| IBIS file stm32mp211_213_215_tfbga289.ibs
[IBIS ver] 5.1
[File name] stm32mp211_213_215_tfbga289.ibs
[File Rev] 0.4
[Date] 09-10-2025
[Source] Data Created at STMicroelectronics
[Notes]  File originated from ELDO simulations.
[Disclaimer]  This information is for modeling purpose only and is
   not guaranted. The information is subject to change without
   notice.
[Copyright] Copyright 2025 STMicroelectronics Inc.
|   Component stm32mp211_213_215_tfbga289
[Component] stm32mp211_213_215_tfbga289
[Manufacturer] STMicroelectronics
[Package]
| variable   typ   min   max
R_pkg  0  NA  NA
L_pkg  0  NA  NA
C_pkg  0  NA  NA
[Pin]   signal_name   model_name
A1  VSS  gnd
A2  CSI_D1P  DPHY_IBIS_L1
A3  CSI_CKP  DPHY_IBIS_L1
A4  PD11  io8_tt_i3c
A5  PD2  io8_tt
A6  PB7  io8_tt
A7  PD15  io8_tt_i3c
A8  PB10  io8_tt
A9  PE5  io8_tt
A10  PE2  io8_tt
A11  PE7  io8_tt
A12  PE11  io8_tt
A13  PE10  io8_tt
A14  PD13  io8_tt
A15  DDR_DQ11  mal4drv27_PAD
A16  DDR_DQ9  mal4drv27_PAD
A17  VSS  gnd
B1  CSI_D0P  DPHY_IBIS_L1
B2  CSI_D1N  DPHY_IBIS_L1
B3  CSI_CKN  DPHY_IBIS_L1
B4  PD10  io8_tt_i3c
B5  PD3  io8_tt
B6  PD8  io8_tt
B7  PB1  io8_tt
B8  PD0  io8_tt
B9  PE4  io8_tt
B10  PE1  io8_tt
B11  PE6  io8_tt
B12  PE9  io8_tt
B13  PE12  io8_tt
B14  PB12  io8_tt
B15  DDR_DQ10  mal4drv27_PAD
B16  DDR_DQS1N  mal4drv27_PAD
B17  DDR_DQS1P  mal4drv27_PAD
C1  CSI_D0N  DPHY_IBIS_L1
C2  VDDCSI  nc
C3  CSI_REXT  nc
C4  VDDA18CSI  power
C5  PD4  io8_tt
C6  PD1  io8_tt
C7  PB3  io8_tt
C8  PB2  io8_tt
C9  PE3  io8_tt
C10  PE0  io8_tt
C11  PE8  io8_tt
C12  PE13  io8_tt
C13  PD7  io8_tt
C14  PD12  io8_tt
C15  DDR_DQ8  mal4drv27_PAD
C16  DDR_DQ15  mal4drv27_PAD
C17  DDR_DQM1  mal4drv27_PAD
D1  PI6  io8_tt
D2  PG2  io8_tt_i3c
D3  PB15  io8_tt
D4  PI5  io8_tt
D5  PB11  io8_tt
D6  PB5  io8_tt_i3c
D7  PD9  io8_tt
D8  PD6  io8_tt
D9  PD5  io8_tt
D10  VDDIO1  power
D11  PE15  io8_tt
D12  PE14  io8_tt
D13  PB13  io8_tt
D14  PD14  io8_tt
D15  DDR_DQ14  mal4drv27_PAD
D16  DDR_DQ13  mal4drv27_PAD
D17  DDR_DQ12  mal4drv27_PAD
E1  PI1  io8_tt_i3c
E2  PA7  io8_tt
E3  PF5  io8_tt
E4  PI0  io8_tt
E5  PB6  io8_tt
E6  PB9  io8_tt
E7  VDDCORE  nc
E8  VDDIO3  power
E9  VDDIO3  power
E10  VDDIO2  power
E11  VDDCPU  nc
E12  VSS  gnd
E13  VDDA18PLL1  nc
E14  PB14  io8_tt
E15  DDR_RESETN  nc
E16  DDR_A9  mal4drv20_PAD
E17  DDR_A20  mal4drv20_PAD
F1  PG14  io8_tt
F2  PG15  io8_tt
F3  PF6  io8_tt
F4  PI4  io8_tt
F5  VDDA18PLL2  nc
F6  VDDCORE  nc
F7  VSS  gnd
F8  VDDCORE  nc
F9  VSS  gnd
F10  VDDCPU  nc
F11  VSS  gnd
F12  VDDCPU  nc
F13  VSS  gnd
F14  DDR_ZQ  nc
F15  DDR_A0  mal4drv20_PAD
F16  DDR_A11  mal4drv20_PAD
F17  DDR_A21  mal4drv20_PAD
G1  PG12  io8_tt
G2  PG11  io8_tt
G3  PG10  io8_tt
G4  PG9  io8_tt
G5  V08CAP  nc
G6  VSS  gnd
G7  VDDCORE  nc
G8  VSS  gnd
G9  VDDCORE  nc
G10  VSS  gnd
G11  VDDCPU  nc
G12  VSS  gnd
G13  VDDA18DDR  nc
G14  DDR_A7  mal4drv20_PAD
G15  DDR_A1  mal4drv20_PAD
G16  DDR_A10  mal4drv20_PAD
G17  DDR_A22  mal4drv20_PAD
H1  PF11  io8_tt
H2  PA5  io8_tt
H3  PH5  io8_tt
H4  PG8  io8_tt
H5  VBAT  power
H6  VDDCORE  nc
H7  VSS  gnd
H8  VDDCORE  nc
H9  VSS  gnd
H10  VDDCPU  nc
H11  VSS  gnd
H12  VDDQDDR  power
H13  VSS  gnd
H14  DDR_A8  mal4drv20_PAD
H15  DDR_A6  mal4drv20_PAD
H16  DDR_A25  mal4drv20_PAD
H17  DDR_A23  mal4drv20_PAD
J1  PG7  io8_tt
J2  PZ0  io8_tt_i3c_tamp
J3  PZ3  io8_tt_i3c_tamp
J4  PZ1  io8_tt_i3c_tamp
J5  VSSAON  nc
J6  VSS  gnd
J7  VDDCORE  nc
J8  VSS  gnd
J9  VDDCORE  nc
J10  VSS  gnd
J11  VDDCPU  nc
J12  VSS  gnd
J13  VDDQDDR  power
J14  DDR_A3  mal4drv20_PAD
J15  DDR_A26  mal4drv20_PAD
J16  DDR_A5  mal4drv20_PAD
J17  DDR_A13  mal4drv20_PAD
K1  PA10  io8_tt
K2  PF4  io8_tt
K3  PG5  io8_tt
K4  PA0  io8_tt
K5  VDDA18AON  power
K6  VDDCORE  nc
K7  VSS  gnd
K8  VDDCORE  nc
K9  VSS  gnd
K10  VDDCORE  nc
K11  VSS  gnd
K12  VDDQDDR  power
K13  VSS  gnd
K14  DDR_A27  mal4drv20_PAD
K15  DDR_A14  mal4drv20_PAD
K16  DDR_A4  mal4drv20_PAD
K17  DDR_A2  mal4drv20_PAD
L1  PA1  io8_tt_i3c
L2  PF13  io8_tt
L3  PF15  io8_tt
L4  PI8  io8_tt
L5  PG3  io8_tt
L6  VSSA  nc
L7  VDD  power
L8  VSS  gnd
L9  VDD  power
L10  VSS  gnd
L11  VDDCORE  nc
L12  VSS  gnd
L13  VDDQDDR  power
L14  DDR_VREF  nc
L15  DDR_A16  mal4drv20_PAD
L16  DDR_A28  mal4drv20_PAD
L17  DDR_A15  mal4drv20_PAD
M1  PG4  io8_tt
M2  PG13  io8_tt_i3c
M3  PC13  io8_tt
M4  PF10  io8_tt
M5  PF8  io8_tt
M6  VDDA18ADC  power
M7  VSS  gnd
M8  VDD  power
M9  VSS  gnd
M10  VDD  power
M11  VSS  gnd
M12  PF3  io8_tt
M13  PA2  io8_tt_i3c
M14  PA3  io8_tt_i3c
M15  DDR_A31  mal4drv20_PAD
M16  DDR_A17  mal4drv20_PAD
M17  DDR_A29  mal4drv20_PAD
N1  PF12  io8_tt
N2  NJTRST  io8_tt
N3  JTCK_SWCLK  io8_tt
N4  JTMS_SWDIO  io8_tt
N5  PC3  io8_tt
N6  PF7  io8_tt
N7  PC4  io8_tt
N8  PC10  io8_tt
N9  PC0  io8_tt
N10  PH9  io8_tt
N11  PF2  io8_tt_i3c
N12  PH8  io8_tt
N13  PA9  io8_tt
N14  PH4  io8_tt
N15  DDR_A12  mal4drv20_PAD
N16  DDR_A18  mal4drv20_PAD
N17  DDR_A30  mal4drv20_PAD
P1  OSC32_IN  isudq_v18
P2  OSC32_OUT  isudq_v18
P3  JTDI  io8_tt
P4  JTDO_TRACESWO  io8_tt
P5  PC5  io8_tt_i3c
P6  PC6  io8_tt_i3c
P7  PC7  io8_tt
P8  PC9  io8_tt
P9  PA14  io8_tt
P10  PA11  io8_tt
P11  PF0  io8_tt_i3c
P12  PH7  io8_tt
P13  VDDA18USB  power
P14  VDD33USB  power
P15  DDR_DQM0  mal4drv27_PAD
P16  DDR_DQ5  mal4drv27_PAD
P17  DDR_DQ4  mal4drv27_PAD
R1  PWR_CPUON  io8_tt
R2  NRST  nc
R3  PWR_ON  io8_tt
R4  PWR_LP  io8_tt
R5  BOOT3  isudq_tt
R6  PG0  io8_tt_i3c
R7  PC12  io8_tt_i3c
R8  PC8  io8_tt
R9  PA13  io8_tt
R10  PA15  io8_tt_i3c
R11  PH11  io8_tt
R12  PA8  io8_tt_i3c
R13  USBH_HS_TXRTUNE  nc
R14  OTG_TXRTUNE  nc
R15  DDR_DQ3  mal4drv27_PAD
R16  DDR_DQ7  mal4drv27_PAD
R17  DDR_DQ6  mal4drv27_PAD
T1  PDR_ON  nc
T2  OSC_IN  isudq_v18
T3  BOOT2  isudq_tt
T4  BOOT0  isudq_tt
T5  VREFN  nc
T6  ANA0  nc
T7  PF9  io8_tt
T8  PF1  io8_tt
T9  PH12  io8_tt
T10  PC1  io8_tt_i3c
T11  PG1  io8_tt_i3c
T12  PA6  io8_tt
T13  USBH_HS_DP  USB2_HS_IBIS
T14  OTG_HSDP  USB2_HS_IBIS
T15  DDR_DQ2  mal4drv27_PAD
T16  DDR_DQS0N  mal4drv27_PAD
T17  DDR_DQS0P  mal4drv27_PAD
U1  VSS  gnd
U2  OSC_OUT  isudq_v18
U3  BOOT1  isudq_tt
U4  NRSTC1MS  io8_tt
U5  VREFP  nc
U6  ANA1  nc
U7  PC11  io8_tt
U8  PC2  io8_tt
U9  PH13  io8_tt
U10  PH10  io8_tt
U11  PA12  io8_tt_i3c
U12  PA4  io8_tt
U13  USBH_HS_DM  USB2_HS_IBIS
U14  OTG_HSDM  USB2_HS_IBIS
U15  DDR_DQ1  mal4drv27_PAD
U16  DDR_DQ0  mal4drv27_PAD
U17  VSS  gnd
[Package Model]   503-fctfbga-14x14-289-240814
[Pin Mapping]   pulldown_ref   pullup_ref   | Comment
A1  gnd  nc
A2  gnd  VDDA18CSI
A3  gnd  VDDA18CSI
A4  gnd  vddio3
A5  gnd  vddio3
A6  gnd  vdd
A7  gnd  vdd
A8  gnd  vdd
A9  gnd  vddio1
A10  gnd  vddio1
A11  gnd  vddio1
A12  gnd  vddio2
A13  gnd  vddio2
A14  gnd  vdd
A15  gnd  vddqddr
A16  gnd  vddqddr
A17  gnd  nc
B1  gnd  VDDA18CSI
B2  gnd  VDDA18CSI
B3  gnd  VDDA18CSI
B4  gnd  vddio3
B5  gnd  vddio3
B6  gnd  vddio3
B7  gnd  vdd
B8  gnd  vddio3
B9  gnd  vddio1
B10  gnd  vddio1
B11  gnd  vddio1
B12  gnd  vddio1
B13  gnd  vddio2
B14  gnd  vdd
B15  gnd  vddqddr
B16  gnd  vddqddr
B17  gnd  vddqddr
C1  gnd  VDDA18CSI
C2  nc  nc
C3  nc  nc
C4  nc  VDDA18CSI
C5  gnd  vddio3
C6  gnd  vddio3
C7  gnd  vdd
C8  gnd  vdd
C9  gnd  vddio1
C10  gnd  vddio1
C11  gnd  vddio1
C12  gnd  vddio2
C13  gnd  vddio3
C14  gnd  vdd
C15  gnd  vddqddr
C16  gnd  vddqddr
C17  gnd  vddqddr
D1  gnd  vdd
D2  gnd  vdd
D3  gnd  vdd
D4  gnd  vdd
D5  gnd  vdd
D6  gnd  vdd
D7  gnd  vddio3
D8  gnd  vddio3
D9  gnd  vddio3
D10  nc  vddio1
D11  gnd  vddio2
D12  gnd  vddio2
D13  gnd  vdd
D14  gnd  vdd
D15  gnd  vddqddr
D16  gnd  vddqddr
D17  gnd  vddqddr
E1  gnd  vdd
E2  gnd  vdd
E3  gnd  vdd
E4  gnd  vdd
E5  gnd  vdd
E6  gnd  vdd
E7  nc  nc
E8  nc  vddio3
E9  nc  vddio3
E10  nc  vddio2
E11  nc  nc
E12  gnd  nc
E13  nc  nc
E14  gnd  vdd
E15  nc  nc
E16  gnd  vddqddr
E17  gnd  vddqddr
F1  gnd  vdd
F2  gnd  vdd
F3  gnd  vdd
F4  gnd  vdd
F5  nc  nc
F6  nc  nc
F7  gnd  nc
F8  nc  nc
F9  gnd  nc
F10  nc  nc
F11  gnd  nc
F12  nc  nc
F13  gnd  nc
F14  nc  nc
F15  gnd  vddqddr
F16  gnd  vddqddr
F17  gnd  vddqddr
G1  gnd  vdd
G2  gnd  vdd
G3  gnd  vdd
G4  gnd  vdd
G5  nc  nc
G6  gnd  nc
G7  nc  nc
G8  gnd  nc
G9  nc  nc
G10  gnd  nc
G11  nc  nc
G12  gnd  nc
G13  nc  nc
G14  gnd  vddqddr
G15  gnd  vddqddr
G16  gnd  vddqddr
G17  gnd  vddqddr
H1  gnd  vdd
H2  gnd  vdd
H3  gnd  vdd
H4  gnd  vdd
H5  nc  vsw
H6  nc  nc
H7  gnd  nc
H8  nc  nc
H9  gnd  nc
H10  nc  nc
H11  gnd  nc
H12  nc  vddqddr
H13  gnd  nc
H14  gnd  vddqddr
H15  gnd  vddqddr
H16  gnd  vddqddr
H17  gnd  vddqddr
J1  gnd  vdd
J2  gnd  vdd  | Depending on IO usage
| J2  gnd  vsw  | Depending on IO usage
J3  gnd  vdd  | Depending on IO usage
| J3  gnd  vsw  | Depending on IO usage
J4  gnd  vdd  | Depending on IO usage
| J4  gnd  vsw  | Depending on IO usage
J5  nc  nc
J6  gnd  nc
J7  nc  nc
J8  gnd  nc
J9  nc  nc
J10  gnd  nc
J11  nc  nc
J12  gnd  nc
J13  nc  vddqddr
J14  gnd  vddqddr
J15  gnd  vddqddr
J16  gnd  vddqddr
J17  gnd  vddqddr
K1  gnd  vdd
K2  gnd  vdd
K3  gnd  vdd
K4  gnd  vdd
K5  nc  vdda18aon
K6  nc  nc
K7  gnd  nc
K8  nc  nc
K9  gnd  nc
K10  nc  nc
K11  gnd  nc
K12  nc  vddqddr
K13  gnd  nc
K14  gnd  vddqddr
K15  gnd  vddqddr
K16  gnd  vddqddr
K17  gnd  vddqddr
L1  gnd  vdd
L2  gnd  vdd
L3  gnd  vdd
L4  gnd  vdd
L5  gnd  vdd
L6  nc  nc
L7  nc  vdd
L8  gnd  nc
L9  nc  vdd
L10  gnd  nc
L11  nc  nc
L12  gnd  nc
L13  nc  vddqddr
L14  nc  nc
L15  gnd  vddqddr
L16  gnd  vddqddr
L17  gnd  vddqddr
M1  gnd  vdd
M2  gnd  vdd
M3  gnd  vdd  | Depending on IO usage
| M3  gnd  vsw  | Depending on IO usage
M4  gnd  vdd
M5  gnd  vdd
M6  nc  vdda18adc
M7  gnd  nc
M8  nc  vdd
M9  gnd  nc
M10  nc  vdd
M11  gnd  nc
M12  gnd  vdd
M13  gnd  vdd
M14  gnd  vdd
M15  gnd  vddqddr
M16  gnd  vddqddr
M17  gnd  vddqddr
N1  gnd  vdd
N2  gnd  vdd
N3  gnd  vdd
N4  gnd  vdd
N5  gnd  vdd
N6  gnd  vdd
N7  gnd  vdd
N8  gnd  vdd
N9  gnd  vdd
N10  gnd  vdd
N11  gnd  vdd
N12  gnd  vdd
N13  gnd  vdd
N14  gnd  vdd
N15  gnd  vddqddr
N16  gnd  vddqddr
N17  gnd  vddqddr
P1  gnd  vdd  | Depending on IO usage
| P1  gnd  vsw  | Depending on IO usage
P2  gnd  vdd  | Depending on IO usage
| P2  gnd  vsw  | Depending on IO usage
P3  gnd  vdd
P4  gnd  vdd
P5  gnd  vdd
P6  gnd  vdd
P7  gnd  vdd
P8  gnd  vdd
P9  gnd  vdd
P10  gnd  vdd
P11  gnd  vdd
P12  gnd  vdd
P13  nc  vdda18usb
P14  nc  VDD33USB
P15  gnd  vddqddr
P16  gnd  vddqddr
P17  gnd  vddqddr
R1  gnd  vdd
R2  nc  nc
R3  gnd  vdd
R4  gnd  vdd
R5  gnd  vdd
R6  gnd  vdd
R7  gnd  vdd
R8  gnd  vdd
R9  gnd  vdd
R10  gnd  vdd
R11  gnd  vdd
R12  gnd  vdd
R13  nc  nc
R14  nc  nc
R15  gnd  vddqddr
R16  gnd  vddqddr
R17  gnd  vddqddr
T1  nc  nc
T2  gnd  vdda18aon
T3  gnd  vdd
T4  gnd  vdd
T5  nc  nc
T6  nc  nc
T7  gnd  vdd
T8  gnd  vdd
T9  gnd  vdd
T10  gnd  vdd
T11  gnd  vdd
T12  gnd  vdd
T13  gnd  VDD33USB
T14  gnd  VDD33USB
T15  gnd  vddqddr
T16  gnd  vddqddr
T17  gnd  vddqddr
U1  gnd  nc
U2  gnd  vdda18aon
U3  gnd  vdd
U4  gnd  vdd
U5  nc  nc
U6  nc  nc
U7  gnd  vdd
U8  gnd  vdd
U9  gnd  vdd
U10  gnd  vdd
U11  gnd  vdd
U12  gnd  vdd
U13  gnd  VDD33USB
U14  gnd  VDD33USB
U15  gnd  vddqddr
U16  gnd  vddqddr
U17  gnd  nc
[Diff Pin]  inv_pin  vdiff  tdelay_typ  tdelay_min  tdelay_max
B3  A3  NA  NA  NA  NA
C1  B1  NA  NA  NA  NA
B2  A2  NA  NA  NA  NA
T17  T16  NA  NA  NA  NA
B17  B16  NA  NA  NA  NA
T13  U13  NA  NA  NA  NA   |USBH_HS_DP _DM
T14  U14  NA  NA  NA  NA   |USBH_HS_DP _DM
K16  J16  NA  NA  NA  NA
[Model Selector] USB2_HS_IBIS
USB2_HSRX   USB2 HSRX model
USB2_HSTX_00_0_01_0011_11   TuningBits_AMP_PULSE_RISE_REF_XV=00_0_01_0011_11
USB2_HSTX_00_0_10_0101_11   TuningBits_AMP_PULSE_RISE_REF_XV=00_0_10_0101_11
USB2_HSTX_00_0_11_0111_11   TuningBits_AMP_PULSE_RISE_REF_XV=00_0_11_0111_11
USB2_HSTX_00_1_01_0011_11   TuningBits_AMP_PULSE_RISE_REF_XV=00_1_01_0011_11
USB2_HSTX_00_1_10_0101_11   TuningBits_AMP_PULSE_RISE_REF_XV=00_1_10_0101_11
USB2_HSTX_00_1_11_0111_11   TuningBits_AMP_PULSE_RISE_REF_XV=00_1_11_0111_11
USB2_HSTX_01_0_01_0011_11   TuningBits_AMP_PULSE_RISE_REF_XV=01_0_01_0011_11
USB2_HSTX_01_0_10_0101_11   TuningBits_AMP_PULSE_RISE_REF_XV=01_0_10_0101_11
USB2_HSTX_01_0_11_0111_11   TuningBits_AMP_PULSE_RISE_REF_XV=01_0_11_0111_11
USB2_HSTX_01_1_01_0011_11   TuningBits_AMP_PULSE_RISE_REF_XV=01_1_01_0011_11
USB2_HSTX_01_1_10_0101_11   TuningBits_AMP_PULSE_RISE_REF_XV=01_1_10_0101_11
USB2_HSTX_01_1_11_0111_11   TuningBits_AMP_PULSE_RISE_REF_XV=01_1_11_0111_11
USB2_HSTX_10_0_01_0011_11   TuningBits_AMP_PULSE_RISE_REF_XV=10_0_01_0011_11
USB2_HSTX_10_0_10_0101_11   TuningBits_AMP_PULSE_RISE_REF_XV=10_0_10_0101_11
USB2_HSTX_10_0_11_0111_11   TuningBits_AMP_PULSE_RISE_REF_XV=10_0_11_0111_11
USB2_HSTX_10_1_01_0011_11   TuningBits_AMP_PULSE_RISE_REF_XV=10_1_01_0011_11
USB2_HSTX_10_1_10_0101_11   TuningBits_AMP_PULSE_RISE_REF_XV=10_1_10_0101_11
USB2_HSTX_10_1_11_0111_11   TuningBits_AMP_PULSE_RISE_REF_XV=10_1_11_0111_11
[Model Selector] DPHY_IBIS_L1
DPHY_RX_2P5G_L1   DPHY HSRX model at 2.5Gbps for lane 1
DPHY_RX_1P5G_L1   DPHY HSRX model at 1.5Gbps for lane 1
[Model Selector] io8_tt
io8_tt_ls_3v3 "GPIO - 3V tolerant - low speed - 3.3V range"
io8_tt_ms_3v3 "GPIO - 3V tolerant - med speed - 3.3V range"
io8_tt_fs_3v3 "GPIO - 3V tolerant - fast speed - 3.3V range"
io8_tt_hs_3v3 "GPIO - 3V tolerant - high speed - 3.3V range"
io8_tt_hslv_ls_1v8 "GPIO low voltage optimization - 3V tolerant - low speed - 1.8V range"
io8_tt_hslv_ms_1v8 "GPIO low voltage optimization - 3V tolerant - med speed - 1.8V range"
io8_tt_hslv_fs_1v8 "GPIO low voltage optimization - 3V tolerant - fast speed - 1.8V range"
io8_tt_hslv_hs_1v8 "GPIO low voltage optimization - 3V tolerant - high speed - 1.8V range"
[Model Selector] io8_tt_i3c
io8_tt_ls_3v3 "GPIO - 3V tolerant - low speed - 3.3V range"
io8_tt_ms_3v3 "GPIO - 3V tolerant - med speed - 3.3V range"
io8_tt_fs_3v3 "GPIO - 3V tolerant - fast speed - 3.3V range"
io8_tt_hs_3v3 "GPIO - 3V tolerant - high speed - 3.3V range"
io8_tt_hslv_ls_1v8 "GPIO low voltage optimization - 3V tolerant - low speed - 1.8V range"
io8_tt_hslv_ms_1v8 "GPIO low voltage optimization - 3V tolerant - med speed - 1.8V range"
io8_tt_hslv_fs_1v8 "GPIO low voltage optimization - 3V tolerant - fast speed - 1.8V range"
io8_tt_hslv_hs_1v8 "GPIO low voltage optimization - 3V tolerant - high speed - 1.8V range"
io8_tt_i3c_ls_3v3 "GPIO with I3C open-drain - 3V tolerant - low speed - 3.3V range"
io8_tt_i3c_ms_3v3 "GPIO with I3C open-drain - 3V tolerant - med speed - 3.3V range"
io8_tt_i3c_fs_3v3 "GPIO with I3C open-drain - 3V tolerant - fast speed - 3.3V range"
io8_tt_i3c_hs_3v3 "GPIO with I3C open-drain - 3V tolerant - high speed - 3.3V range"
io8_tt_hslv_i3c_ls_1v8 "GPIO low voltage optimization with I3C open-drain - 3V tolerant - low speed - 1.8V range"
io8_tt_hslv_i3c_ms_1v8 "GPIO low voltage optimization with I3C open-drain - 3V tolerant - med speed - 1.8V range"
io8_tt_hslv_i3c_fs_1v8 "GPIO low voltage optimization with I3C open-drain - 3V tolerant - fast speed - 1.8V range"
io8_tt_hslv_i3c_hs_1v8 "GPIO low voltage optimization with I3C open-drain - 3V tolerant - high speed - 1.8V range"
io8_tt_i3c_fmp_3v3 "GPIO with I3C fm+ open-drain - 3V tolerant - 3.3V range"
[Model Selector] io8_tt_i3c_tamp
io8_tt_ls_3v3 "GPIO - 3V tolerant - low speed - 3.3V range"
io8_tt_ms_3v3 "GPIO - 3V tolerant - med speed - 3.3V range"
io8_tt_fs_3v3 "GPIO - 3V tolerant - fast speed - 3.3V range"
io8_tt_hs_3v3 "GPIO - 3V tolerant - high speed - 3.3V range"
io8_tt_hslv_ls_1v8 "GPIO low voltage optimization - 3V tolerant - low speed - 1.8V range"
io8_tt_hslv_ms_1v8 "GPIO low voltage optimization - 3V tolerant - med speed - 1.8V range"
io8_tt_hslv_fs_1v8 "GPIO low voltage optimization - 3V tolerant - fast speed - 1.8V range"
io8_tt_hslv_hs_1v8 "GPIO low voltage optimization - 3V tolerant - high speed - 1.8V range"
io8_tt_i3c_ls_3v3 "GPIO with I3C open-drain - 3V tolerant - low speed - 3.3V range"
io8_tt_i3c_ms_3v3 "GPIO with I3C open-drain - 3V tolerant - med speed - 3.3V range"
io8_tt_i3c_fs_3v3 "GPIO with I3C open-drain - 3V tolerant - fast speed - 3.3V range"
io8_tt_i3c_hs_3v3 "GPIO with I3C open-drain - 3V tolerant - high speed - 3.3V range"
io8_tt_hslv_i3c_ls_1v8 "GPIO low voltage optimization with I3C open-drain - 3V tolerant - low speed - 1.8V range"
io8_tt_hslv_i3c_ms_1v8 "GPIO low voltage optimization with I3C open-drain - 3V tolerant - med speed - 1.8V range"
io8_tt_hslv_i3c_fs_1v8 "GPIO low voltage optimization with I3C open-drain - 3V tolerant - fast speed - 1.8V range"
io8_tt_hslv_i3c_hs_1v8 "GPIO low voltage optimization with I3C open-drain - 3V tolerant - high speed - 1.8V range"
io8_tt_i3c_fmp_3v3 "GPIO with I3C fm+ open-drain - 3V tolerant - 3.3V range"
io8_tt_tamp_3v3 "IO tamper - 3V tolerant - 3.3V range"
io8_tt_tamp_1v8 "IO tamper - 3V tolerant - 1.8V range"
[Model Selector] isudq_tt
isudq_tt_3v3 "Input Buffer - 3V tolerant - 3.3V range"
isudq_tt_1v8 "Input Buffer - 3V tolerant - 1.8V range"
|[Model Selector] isudq_v18
|isudq_v18_1v8 "Input Buffer - 1.8V range "
[Model Selector]   mal4drv20_PAD
mal4drv20_d3l_40   DDR3L mal4drv20 cell  Z0=40-Ohm Driver
mal4drv20_d3l_60   DDR3L mal4drv20 cell  Z0=60-Ohm Driver
mal4drv20_d3l_120   DDR3L mal4drv20 cell  Z0=120-Ohm Driver
mal4drv20_d3_20   DDR3 mal4drv20 cell  Z0=20-Ohm Driver
mal4drv20_d3_24   DDR3 mal4drv20 cell  Z0=24-Ohm Driver
mal4drv20_d3_30   DDR3 mal4drv20 cell  Z0=30-Ohm Driver
mal4drv20_d3_40   DDR3 mal4drv20 cell  Z0=40-Ohm Driver
mal4drv20_d3_60   DDR3 mal4drv20 cell  Z0=60-Ohm Driver
mal4drv20_d4_20   DDR4 mal4drv20 cell  Z0=20-Ohm Driver
mal4drv20_d4_24   DDR4 mal4drv20 cell  Z0=24-Ohm Driver
mal4drv20_d4_30   DDR4 mal4drv20 cell  Z0=30-Ohm Driver
mal4drv20_d4_40   DDR4 mal4drv20 cell  Z0=40-Ohm Driver
mal4drv20_d4_60   DDR4 mal4drv20 cell  Z0=60-Ohm Driver
mal4drv20_dl4_20   LPDDR4 mal4drv20 cell  Z0=20-Ohm Driver
mal4drv20_dl4_24   LPDDR4 mal4drv20 cell  Z0=24-Ohm Driver
mal4drv20_dl4_30   LPDDR4 mal4drv20 cell  Z0=30-Ohm Driver
mal4drv20_dl4_40   LPDDR4 mal4drv20 cell  Z0=40-Ohm Driver
mal4drv20_dl4_60   LPDDR4 mal4drv20 cell  Z0=60-Ohm Driver
[Model Selector]   mal4drv27_PAD
mal4drv27_d3l_40   DDR3L mal4drv27 cell  Z0=40-Ohm Driver
mal4drv27_d3l_48   DDR3L mal4drv27 cell  Z0=48-Ohm Driver
mal4drv27_d3l_60   DDR3L mal4drv27 cell  Z0=60-Ohm Driver
mal4drv27_d3l_80   DDR3L mal4drv27 cell  Z0=80-Ohm Driver
mal4drv27_d3l_120   DDR3L mal4drv27 cell  Z0=120-Ohm Driver
mal4drv27_d3l_240   DDR3L mal4drv27 cell  Z0=240-Ohm Driver
mal4drv27_d3l_odt120   DDR3L mal4drv27 cell 120-Ohm ODT Receiver
mal4drv27_d3l_odt60   DDR3L mal4drv27 cell 60-Ohm ODT Receiver
mal4drv27_d3l_odtoff   DDR3L mal4drv27 cell ODT OFF Receiver
mal4drv27_d3_28   DDR3 mal4drv27 cell  Z0=28-Ohm Driver
mal4drv27_d3_34   DDR3 mal4drv27 cell  Z0=34-Ohm Driver
mal4drv27_d3_40   DDR3 mal4drv27 cell  Z0=40-Ohm Driver
mal4drv27_d3_53   DDR3 mal4drv27 cell  Z0=53-Ohm Driver
mal4drv27_d3_odt120   DDR3 mal4drv27 cell 120-Ohm ODT Receiver
mal4drv27_d3_odt60   DDR3 mal4drv27 cell 60-Ohm ODT Receiver
mal4drv27_d4_28   DDR4 mal4drv27 cell  Z0=28-Ohm Driver
mal4drv27_d4_34   DDR4 mal4drv27 cell  Z0=34-Ohm Driver
mal4drv27_d4_40   DDR4 mal4drv27 cell  Z0=40-Ohm Driver
mal4drv27_d4_53   DDR4 mal4drv27 cell  Z0=53-Ohm Driver
mal4drv27_d4_odt120   DDR4 mal4drv27 cell 120-Ohm ODT Receiver
mal4drv27_d4_odt240   DDR4 mal4drv27 cell 240-Ohm ODT Receiver
mal4drv27_d4_odt48   DDR4 mal4drv27 cell 48-Ohm ODT Receiver
mal4drv27_d4_odt60   DDR4 mal4drv27 cell 60-Ohm ODT Receiver
mal4drv27_d4_odt80   DDR4 mal4drv27 cell 80-Ohm ODT Receiver
mal4drv27_dl4_28   LPDDR4 mal4drv27 cell  Z0=28-Ohm Driver
mal4drv27_dl4_34   LPDDR4 mal4drv27 cell  Z0=34-Ohm Driver
mal4drv27_dl4_40   LPDDR4 mal4drv27 cell  Z0=40-Ohm Driver
mal4drv27_dl4_53   LPDDR4 mal4drv27 cell  Z0=53-Ohm Driver
mal4drv27_dl4_odt48   LPDDR4 mal4drv27 cell 48-Ohm ODT Receiver
mal4drv27_dl4_odt60   LPDDR4 mal4drv27 cell 60-Ohm ODT Receiver
[Define Package Model]  503-fctfbga-14x14-289-240814
[Manufacturer]  unknown
[OEM]  unknown
[Description]  unknown
[Number Of Pins]  235
[Pin Numbers]
| Pin Name Terminal   Net Name   Starting Node   Ending Node
T6 | ANA0
U6 | ANA1
T4 | BOOT0
U3 | BOOT1
T3 | BOOT2
R5 | BOOT3
B3 | CSI_CKN
A3 | CSI_CKP
C1 | CSI_D0N
B1 | CSI_D0P
B2 | CSI_D1N
A2 | CSI_D1P
C3 | CSI_REXT
F15 | DDR_A0
G15 | DDR_A1
K17 | DDR_A2
J14 | DDR_A3
K16 | DDR_A4
J16 | DDR_A5
H15 | DDR_A6
G14 | DDR_A7
H14 | DDR_A8
E16 | DDR_A9
G16 | DDR_A10
F16 | DDR_A11
N15 | DDR_A12
J17 | DDR_A13
K15 | DDR_A14
L17 | DDR_A15
L15 | DDR_A16
M16 | DDR_A17
N16 | DDR_A18
E17 | DDR_A20
F17 | DDR_A21
G17 | DDR_A22
H17 | DDR_A23
H16 | DDR_A25
J15 | DDR_A26
K14 | DDR_A27
L16 | DDR_A28
M17 | DDR_A29
N17 | DDR_A30
M15 | DDR_A31
U16 | DDR_DQ0
U15 | DDR_DQ1
T15 | DDR_DQ2
R15 | DDR_DQ3
P17 | DDR_DQ4
P16 | DDR_DQ5
R17 | DDR_DQ6
R16 | DDR_DQ7
C15 | DDR_DQ8
A16 | DDR_DQ9
B15 | DDR_DQ10
A15 | DDR_DQ11
D17 | DDR_DQ12
D16 | DDR_DQ13
D15 | DDR_DQ14
C16 | DDR_DQ15
P15 | DDR_DQM0
C17 | DDR_DQM1
T16 | DDR_DQS0N
T17 | DDR_DQS0P
B16 | DDR_DQS1N
B17 | DDR_DQS1P
E15 | DDR_RESETN
L14 | DDR_VREF
F14 | DDR_ZQ
N3 | JTCK_SWCLK
P3 | JTDI
P4 | JTDO_TRACESWO
N4 | JTMS_SWDIO
N2 | NJTRST
R2 | NRST
U4 | NRSTC1MS
P1 | OSC32_IN
P2 | OSC32_OUT
T2 | OSC_IN
U2 | OSC_OUT
U14 | OTG_HSDM
T14 | OTG_HSDP
R14 | OTG_TXRTUNE
K4 | PA0
L1 | PA1
M13 | PA2
M14 | PA3
U12 | PA4
H2 | PA5
T12 | PA6
E2 | PA7
R12 | PA8
N13 | PA9
K1 | PA10
P10 | PA11
U11 | PA12
R9 | PA13
P9 | PA14
R10 | PA15
B7 | PB1
C8 | PB2
C7 | PB3
D6 | PB5
E5 | PB6
A6 | PB7
E6 | PB9
A8 | PB10
D5 | PB11
B14 | PB12
D13 | PB13
E14 | PB14
D3 | PB15
N9 | PC0
T10 | PC1
U8 | PC2
N5 | PC3
N7 | PC4
P5 | PC5
P6 | PC6
P7 | PC7
R8 | PC8
P8 | PC9
N8 | PC10
U7 | PC11
R7 | PC12
M3 | PC13
B8 | PD0
C6 | PD1
A5 | PD2
B5 | PD3
C5 | PD4
D9 | PD5
D8 | PD6
C13 | PD7
B6 | PD8
D7 | PD9
B4 | PD10
A4 | PD11
C14 | PD12
A14 | PD13
D14 | PD14
A7 | PD15
T1 | PDR_ON
C10 | PE0
B10 | PE1
A10 | PE2
C9 | PE3
B9 | PE4
A9 | PE5
B11 | PE6
A11 | PE7
C11 | PE8
B12 | PE9
A13 | PE10
A12 | PE11
B13 | PE12
C12 | PE13
D12 | PE14
D11 | PE15
P11 | PF0
T8 | PF1
N11 | PF2
M12 | PF3
K2 | PF4
E3 | PF5
F3 | PF6
N6 | PF7
M5 | PF8
T7 | PF9
M4 | PF10
H1 | PF11
N1 | PF12
L2 | PF13
L3 | PF15
R6 | PG0
T11 | PG1
D2 | PG2
L5 | PG3
M1 | PG4
K3 | PG5
J1 | PG7
H4 | PG8
G4 | PG9
G3 | PG10
G2 | PG11
G1 | PG12
M2 | PG13
F1 | PG14
F2 | PG15
N14 | PH4
H3 | PH5
P12 | PH7
N12 | PH8
N10 | PH9
U10 | PH10
R11 | PH11
T9 | PH12
U9 | PH13
E4 | PI0
E1 | PI1
F4 | PI4
D4 | PI5
D1 | PI6
L4 | PI8
R1 | PWR_CPUON
R4 | PWR_LP
R3 | PWR_ON
J2 | PZ0
J4 | PZ1
J3 | PZ3
U13 | USBH_HS_DM
T13 | USBH_HS_DP
R13 | USBH_HS_TXRTUNE
G5 | V08CAP
H5 | VBAT
P14 | VDD33USB
L7 | VDD
M6 | VDDA18ADC
K5 | VDDA18AON
C4 | VDDA18CSI
G13 | VDDA18DDR
E13 | VDDA18PLL1
F5 | VDDA18PLL2
P13 | VDDA18USB
E7 | VDDCORE
E11 | VDDCPU
C2 | VDDCSI
D10 | VDDIO1
E10 | VDDIO2
E8 | VDDIO3
H12 | VDDQDDR
T5 | VREFN
U5 | VREFP
A1 | VSS
L6 | VSSA
J5 | VSSAON
|[Merged Pins]  L7
|L9  |  VDD
|M8  |  VDD
|M10  |  VDD
|[Merged Pins]  E7
|F6  |  VDDCORE
|F8  |  VDDCORE
|G7  |  VDDCORE
|G9  |  VDDCORE
|H6  |  VDDCORE
|H8  |  VDDCORE
|J7  |  VDDCORE
|J9  |  VDDCORE
|K6  |  VDDCORE
|K8  |  VDDCORE
|K10  |  VDDCORE
|L11  |  VDDCORE
|[Merged Pins]  E11
|F10  |  VDDCPU
|F12  |  VDDCPU
|G11  |  VDDCPU
|H10  |  VDDCPU
|J11  |  VDDCPU
|[Merged Pins]  E8
|E9  |  VDDIO3
|[Merged Pins]  H12
|J13  |  VDDQDDR
|K12  |  VDDQDDR
|L13  |  VDDQDDR
|[Merged Pins]  A1
|A17  |  VSS
|E12  |  VSS
|F7  |  VSS
|F9  |  VSS
|F11  |  VSS
|F13  |  VSS
|G6  |  VSS
|G8  |  VSS
|G10  |  VSS
|G12  |  VSS
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[Model Data]
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[End Model Data]
[End Package Model]
|End [Component]
| Models and submodels in the file (91): USB2_HSRX (Input), USB2_HSTX_00_0_01_0011_11 (Output), USB2_HSTX_00_0_10_0101_11 (Output), USB2_HSTX_00_0_11_0111_11 (Output), USB2_HSTX_00_1_01_0011_11 (Output), USB2_HSTX_00_1_10_0101_11 (Output), USB2_HSTX_00_1_11_0111_11 (Output), USB2_HSTX_01_0_01_0011_11 (Output), USB2_HSTX_01_0_10_0101_11 (Output), USB2_HSTX_01_0_11_0111_11 (Output), USB2_HSTX_01_1_01_0011_11 (Output), USB2_HSTX_01_1_10_0101_11 (Output), USB2_HSTX_01_1_11_0111_11 (Output), USB2_HSTX_10_0_01_0011_11 (Output), USB2_HSTX_10_0_10_0101_11 (Output), USB2_HSTX_10_0_11_0111_11 (Output), USB2_HSTX_10_1_01_0011_11 (Output), USB2_HSTX_10_1_10_0101_11 (Output), USB2_HSTX_10_1_11_0111_11 (Output), DPHY_RX_1P5G_L1 (Input), DPHY_RX_2P5G_L1 (Input), mal4drv20_d3_20 (I/O), mal4drv20_d3_24 (I/O), mal4drv20_d3_30 (I/O), mal4drv20_d3_40 (I/O), mal4drv20_d3_60 (I/O), mal4drv20_d4_20 (I/O), mal4drv20_d4_24 (I/O), mal4drv20_d4_30 (I/O), mal4drv20_d4_40 (I/O), mal4drv20_d4_60 (I/O), mal4drv20_dl4_20 (I/O), mal4drv20_dl4_24 (I/O), mal4drv20_dl4_30 (I/O), mal4drv20_dl4_40 (I/O), mal4drv20_dl4_60 (I/O), mal4drv27_d3_28 (I/O), mal4drv27_d3_34 (I/O), mal4drv27_d3_40 (I/O), mal4drv27_d3_53 (I/O), mal4drv27_d3_odt120 (Input), mal4drv27_d3_odt60 (Input), mal4drv27_dl4_28 (I/O), mal4drv27_dl4_34 (I/O), mal4drv27_dl4_40 (I/O), mal4drv27_dl4_53 (I/O), mal4drv27_dl4_odt48 (Input), mal4drv27_dl4_odt60 (Input), mal4drv27_d4_28 (I/O), mal4drv27_d4_34 (I/O), mal4drv27_d4_40 (I/O), mal4drv27_d4_53 (I/O), mal4drv27_d4_odt120 (Input), mal4drv27_d4_odt240 (Input), mal4drv27_d4_odt48 (Input), mal4drv27_d4_odt60 (Input), mal4drv27_d4_odt80 (Input), mal4drv20_d3l_120 (I/O), mal4drv20_d3l_40 (I/O), mal4drv20_d3l_60 (I/O), mal4drv27_d3l_120 (I/O), mal4drv27_d3l_240 (I/O), mal4drv27_d3l_40 (I/O), mal4drv27_d3l_48 (I/O), mal4drv27_d3l_60 (I/O), mal4drv27_d3l_80 (I/O), mal4drv27_d3l_odt120 (Input), mal4drv27_d3l_odt60 (Input), mal4drv27_d3l_odtoff (Input), io8_tt_fs_3v3 (I/O), io8_tt_hs_3v3 (I/O), io8_tt_hslv_fs_1v8 (I/O), io8_tt_hslv_hs_1v8 (I/O), io8_tt_hslv_i3c_fs_1v8 (I/O_open_drain), io8_tt_hslv_i3c_hs_1v8 (I/O_open_drain), io8_tt_hslv_i3c_ls_1v8 (I/O_open_drain), io8_tt_hslv_i3c_ms_1v8 (I/O_open_drain), io8_tt_hslv_ls_1v8 (I/O), io8_tt_hslv_ms_1v8 (I/O), io8_tt_i3c_fmp_3v3 (I/O_open_drain)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
